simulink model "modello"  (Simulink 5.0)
settings: Solver=ode45  StartTime=0.0  StopTime=250  FixedStep=0.1  RelTol=1e-3
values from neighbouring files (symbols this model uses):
  Ct = Ctfe+Ctcu    [Capacita.m]
  Gt = 1/Rt    [Capacita.m]
  Pp = DTreg/Rt    [Capacita.m]

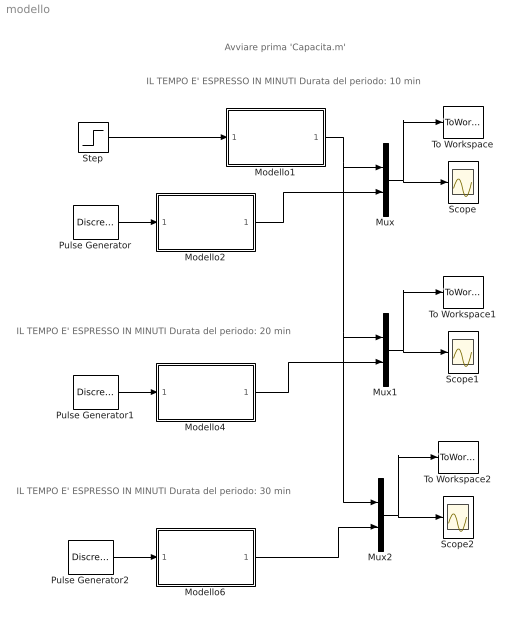
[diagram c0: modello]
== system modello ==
  note: IL TEMPO E' ESPRESSO IN MINUTI Durata del periodo: 10 min
  note: Avviare prima 'Capacita.m'
  note: IL TEMPO E' ESPRESSO IN MINUTI Durata del periodo: 20 min
  note: IL TEMPO E' ESPRESSO IN MINUTI Durata del periodo: 30 min
  Modello1 : Subsystem
  Modello2 : Subsystem
  Modello4 : Subsystem
  Modello6 : Subsystem
  Mux : Mux  Inputs=2
  Mux1 : Mux  Inputs=2
  Mux2 : Mux  Inputs=2
  Pulse Generator : DiscretePulseGenerator  PulseType=Time based  Amplitude=2*Pp  Period=10  PulseWidth=50  SampleTime=10
  Pulse Generator1 : DiscretePulseGenerator  PulseType=Time based  Amplitude=2*Pp  Period=20  PulseWidth=50  SampleTime=10
  Pulse Generator2 : DiscretePulseGenerator  PulseType=Time based  Amplitude=2*Pp  Period=30  PulseWidth=50  SampleTime=10
  Scope : Scope
  Scope1 : Scope
  Scope2 : Scope
  Step : Step  Time=0  After=Pp  SampleTime=0
  To Workspace : ToWorkspace  VariableName=m1  SampleTime=-1  SaveFormat=Array
  To Workspace1 : ToWorkspace  VariableName=m2  SampleTime=-1  SaveFormat=Array
  To Workspace2 : ToWorkspace  VariableName=m3  SampleTime=-1  SaveFormat=Array
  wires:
  Step/1 -> Modello1/1(In1)
  Mux/1 -> To Workspace/1, Scope/1
  Modello1/1(Out1) -> Mux/1, Mux1/1, Mux2/1
  Pulse Generator/1 -> Modello2/1(In1)
  Modello2/1(Out1) -> Mux/2
  Mux1/1 -> Scope1/1, To Workspace1/1
  Pulse Generator1/1 -> Modello4/1(In1)
  Modello4/1(Out1) -> Mux1/2
  Mux2/1 -> To Workspace2/1, Scope2/1
  Pulse Generator2/1 -> Modello6/1(In1)
  Modello6/1(Out1) -> Mux2/2

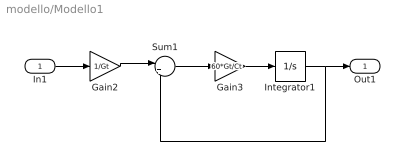
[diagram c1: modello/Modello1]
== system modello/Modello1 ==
  In1 : Inport
  Gain2 : Gain  Gain=1/Gt
  Gain3 : Gain  Gain=60*Gt/Ct
  Integrator1 : Integrator
  Sum1 : Sum  Inputs=|+-
  Out1 : Outport
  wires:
  Gain2/1 -> Sum1/1
  Sum1/1 -> Gain3/1
  Gain3/1 -> Integrator1/1
  Integrator1/1 -> Sum1/2, Out1/1
  In1/1 -> Gain2/1

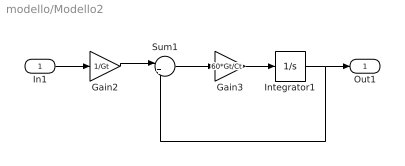
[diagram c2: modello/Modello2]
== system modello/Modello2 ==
  In1 : Inport
  Gain2 : Gain  Gain=1/Gt
  Gain3 : Gain  Gain=60*Gt/Ct
  Integrator1 : Integrator
  Sum1 : Sum  Inputs=|+-
  Out1 : Outport
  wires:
  In1/1 -> Gain2/1
  Integrator1/1 -> Out1/1, Sum1/2
  Gain3/1 -> Integrator1/1
  Sum1/1 -> Gain3/1
  Gain2/1 -> Sum1/1

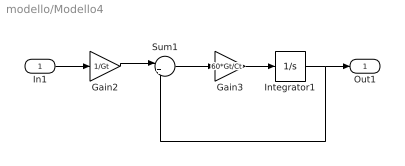
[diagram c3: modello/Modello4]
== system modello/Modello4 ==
  In1 : Inport
  Gain2 : Gain  Gain=1/Gt
  Gain3 : Gain  Gain=60*Gt/Ct
  Integrator1 : Integrator
  Sum1 : Sum  Inputs=|+-
  Out1 : Outport
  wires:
  Gain2/1 -> Sum1/1
  Sum1/1 -> Gain3/1
  Gain3/1 -> Integrator1/1
  Integrator1/1 -> Sum1/2, Out1/1
  In1/1 -> Gain2/1

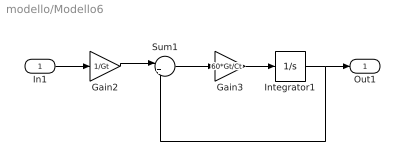
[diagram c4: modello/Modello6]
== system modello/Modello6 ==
  In1 : Inport
  Gain2 : Gain  Gain=1/Gt
  Gain3 : Gain  Gain=60*Gt/Ct
  Integrator1 : Integrator
  Sum1 : Sum  Inputs=|+-
  Out1 : Outport
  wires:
  In1/1 -> Gain2/1
  Integrator1/1 -> Out1/1, Sum1/2
  Gain3/1 -> Integrator1/1
  Sum1/1 -> Gain3/1
  Gain2/1 -> Sum1/1
